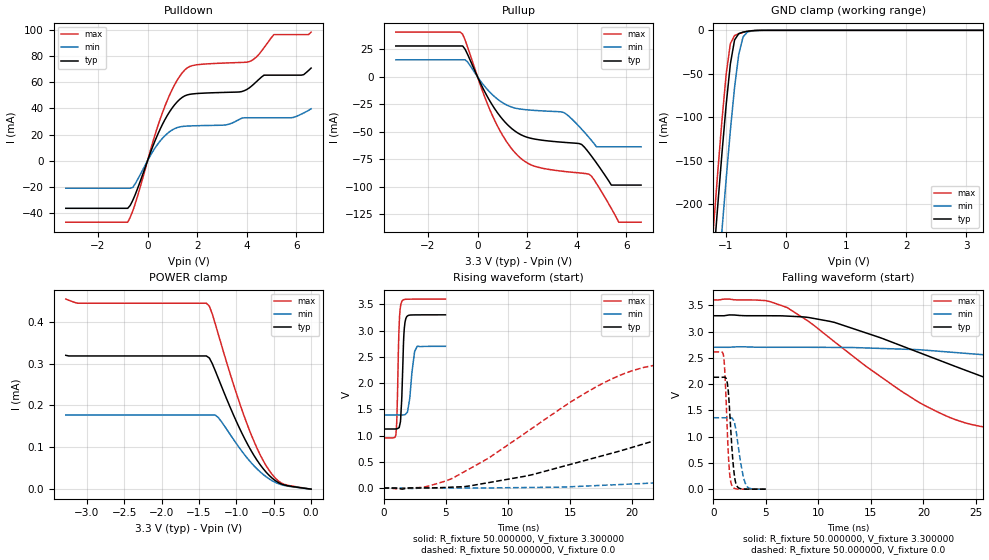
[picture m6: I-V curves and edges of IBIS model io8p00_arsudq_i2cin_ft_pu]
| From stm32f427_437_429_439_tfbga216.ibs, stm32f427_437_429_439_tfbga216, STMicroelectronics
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|   Model io8p00_arsudq_i2cin_ft_pu
[Model]  io8p00_arsudq_i2cin_ft_pu
Model_type I/O
Polarity   Non-Inverting
Enable   Active-Low
Vinl =   0.990000V
Vinh =   2.310000V
Vmeas =  1.650000V
Cref =   50.000000pF
Rref =   100.000000M
Vref =   0.0V
C_comp   2.280000pF   2.217000pF   2.355700pF
[Temperature Range]   25.000000   0.125000k   -40.000000
[Pullup Reference]   3.300000V   2.700000V   3.600000V
[Pulldown Reference]   0.0V   0.0V   0.0V
[POWER Clamp Reference]   3.300000V   2.700000V   3.600000V
[GND Clamp Reference]   0.0V   0.0V   0.0V
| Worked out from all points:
|   slope of the pulldown table from 0 to 0.495 V, typ, clamps not added: 20.9 ohm
|   slope of the pullup table from 0 to 0.495 V, typ, clamps not added: 22.6 ohm
|   GND clamp passes 1 mA (typ) near -0.62 V on its own axis
|   rising waveform, R_fixture 50.000000, V_fixture 3.300000: 20-80 % time 190ps typ, 341ps min, 164ps max; typ from 1.12 V to 3.3 V
|   rising waveform, R_fixture 50.000000, V_fixture 0.0: 20-80 % time 19.7ns typ, 51ns min, 10.4ns max; typ from 0.001 V to 2.13 V
|   falling waveform, R_fixture 50.000000, V_fixture 3.300000: 20-80 % time 18.7ns typ, 37.6ns min, 11.4ns max; typ from 3.3 V to 1.12 V
|   falling waveform, R_fixture 50.000000, V_fixture 0.0: 20-80 % time 433ps typ, 633ps min, 342ps max; typ from 2.13 V to 0.001 V
[Pulldown]
|Voltage   I(typ)   I(min)   I(max)
-3.3V     -36.46mA   -21.09mA   -47.09mA
-800mV    -36.46mA   -21.09mA   -47.09mA
-600mV    -30.5mA    -20.55mA   -38.69mA
700mV     31.4mA     19.11mA    41.71mA
1.2V      45.15mA    25.37mA    61.75mA
1.6V      50.35mA    26.5mA     71.06mA
3.1V      52.28mA    27.26mA    74.76mA
4.1V      55.64mA    32.87mA    75.8mA
4.7V      65.47mA    32.87mA    86.49mA
5.1V      65.47mA    32.87mA    96.56mA
6.2V      65.47mA    35.57mA    96.56mA
6.6V      70.92mA    39.71mA    98.46mA
[Pullup]
|Voltage   I(typ)   I(min)   I(max)
-3.3V     28.01mA    15.42mA    40.63mA
-700mV    28.01mA    15.42mA    40.63mA
-400mV    20.31mA    13.47mA    26.93mA
600mV     -25.77mA   -16.23mA   -35.13mA
1.6V      -50.64mA   -28.8mA    -70.96mA
3.5V      -59.52mA   -32.65mA   -85.91mA
4.2V      -61.43mA   -47.48mA   -87.45mA
4.5V      -69.07mA   -55.12mA   -88.37mA
4.8V      -78.21mA   -63.5mA    -96.83mA
5.4V      -98.3mA    -63.5mA    -119.6mA
5.7V      -98.3mA    -63.5mA    -132mA
6.6V      -98.3mA    -63.5mA    -132mA
[GND_clamp]
|Voltage   I(typ)   I(min)   I(max)
-3.3V     -2.32A     -2.398A    -2.293A
-1.2V     -265.5mA   -356.1mA   -227.2mA
-1.13V    -202.6mA   -292.9mA   -164.1mA
-1.06V    -142.2mA   -231.2mA   -104.1mA
-990mV    -85.98mA   -171.6mA   -50.72mA
-920mV    -38.8mA    -115.5mA   -15.28mA
-850mV    -11.08mA   -65.6mA    -6.001mA
-780mV    -3.782mA   -27.42mA   -3.876mA
-710mV    -2.086mA   -7.69mA    -2.381mA
-640mV    -1.147mA   -2.118mA   -1.22mA
-570mV    -523.9uA   -798.4uA   -476.8uA
3.28V     0A         0A         0A
[POWER_clamp]
|Voltage   I(typ)   I(min)   I(max)
-3.28V    319.9uA    177.1uA    454.3uA
-3.12V    318.3uA    177.1uA    444.3uA
-1.4V     318.3uA    177.1uA    444.3uA
-1.36V    313.4uA    177.1uA    437.2uA
-1.28V    282.3uA    177.1uA    394.1uA
-1.24V    264.6uA    170.9uA    369.7uA
-920mV    131.9uA    89.35uA    187.2uA
-760mV    79.47uA    55.13uA    112.7uA
-640mV    48.78uA    35.04uA    68.06uA
-520mV    26.21uA    20.11uA    35uA
-400mV    12.52uA    10.81uA    14.88uA
0V        0A         0A         0A
[Ramp]
| variable   typ   min   max
dV/dt_r  1.27723/19.71538n   0.81543/51.02379n   1.56688/10.34644n
dV/dt_f  1.30524/18.67597n   0.78396/37.71750n   1.58713/11.33655n
R_load = 50.000000
[Rising Waveform]
R_fixture= 50.000000
V_fixture= 3.300000
V_fixture_min= 2.700000
V_fixture_max= 3.600000
|time   V(typ)   V(min)   V(max)
0s        1.125V     1.393V     954.7mV
1.001ns   1.127V     1.393V     1.027V
1.071ns   1.129V     1.393V     1.309V
1.281ns   1.174V     1.393V     3.222V
1.451ns   1.629V     1.392V     3.542V
1.632ns   2.896V     1.395V     3.589V
1.852ns   3.258V     1.43V      3.596V
2.503ns   3.298V     2.601V     3.599V
2.713ns   3.299V     2.701V     3.599V
4.985ns   3.3V       2.7V       3.6V
[Rising Waveform]
R_fixture= 50.000000
V_fixture= 0.0
V_fixture_min= 0.0
V_fixture_max= 0.0
|time   V(typ)   V(min)   V(max)
0s        1.088mV    1.043mV    1.136mV
5.506ns   17.87mV    2.788mV    181.7mV
11.51ns   231.2mV    10.97mV    1.067V
19.52ns   741.9mV    73.07mV    2.196V
30.53ns   1.49V      220.5mV    2.532V
39.54ns   1.884V     380.3mV    2.581V
52.55ns   2.046V     618.4mV    2.603V
88.59ns   2.123V     1.136V     2.613V
116.6ns   2.129V     1.298V     2.613V
249.2ns   2.13V      1.36V      2.613V
[Falling Waveform]
R_fixture= 50.000000
V_fixture= 3.300000
V_fixture_min= 2.700000
V_fixture_max= 3.600000
|time   V(typ)   V(min)   V(max)
0s        3.3V       2.7V       3.6V
7.007ns   3.293V     2.7V       3.456V
11.51ns   3.174V     2.697V     2.807V
18.02ns   2.72V      2.664V     1.85V
22.52ns   2.375V     2.608V     1.363V
32.03ns   1.696V     2.419V     1.066V
47.05ns   1.271V     2.077V     992.4mV
67.57ns   1.171V     1.667V     964.9mV
85.09ns   1.147V     1.534V     959.3mV
249.2ns   1.125V     1.393V     954.7mV
[Falling Waveform]
R_fixture= 50.000000
V_fixture= 0.0
V_fixture_min= 0.0
V_fixture_max= 0.0
|time   V(typ)   V(min)   V(max)
0s        2.13V      1.36V      2.613V
981ps     2.131V     1.36V      2.506V
1.151ns   2.12V      1.359V     1.94V
1.411ns   1.865V     1.36V      679.8mV
1.542ns   1.481V     1.362V     293mV
1.732ns   855.6mV    1.355V     80.58mV
2.152ns   98.39mV    1.117V     6.19mV
2.823ns   3.622mV    253mV      1.349mV
3.123ns   1.866mV    72.52mV    1.239mV
4.985ns   1.088mV    1.043mV    1.136mV
